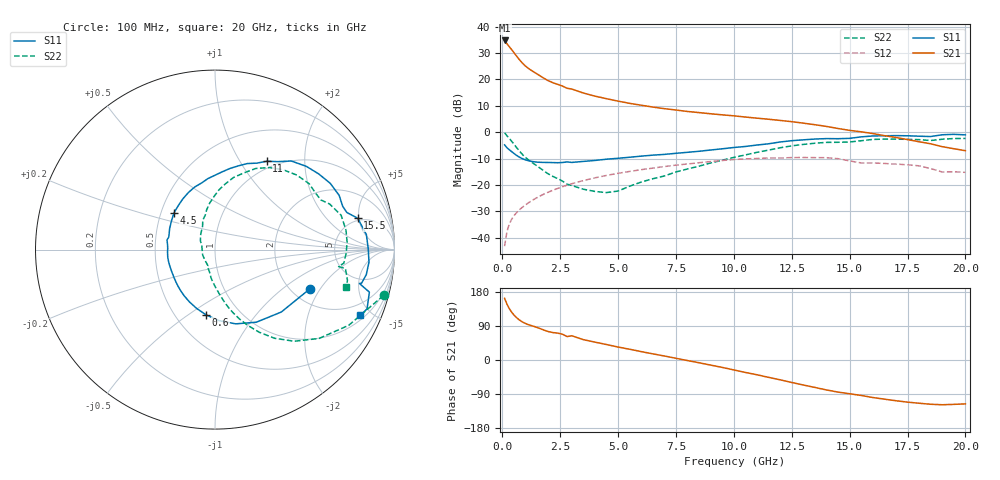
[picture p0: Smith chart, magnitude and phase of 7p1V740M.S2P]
! Infineon Technologies  Discrete & RF Semiconductors
! bfp620
! VCE =  1.7 V,  IC =  40 mA
! Common Emitter S-Parameters:  Sep 2002
# GHz  S  MA  R  50
!  f  S11  S21  S12  S22
! GHz  MAG  ANG  MAG  ANG  MAG  ANG  MAG  ANG
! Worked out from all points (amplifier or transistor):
!   59 points, 100 MHz to 20 GHz, reference 50 ohm
!   highest |S21| = 34.8 dB at 100 MHz (marker M1)
!   |S21| within 3 dB of that: start of sweep to 361.1 MHz
!   unconditionally stable (mu >= 1): 2.754 GHz to 2.94 GHz; 3.04 GHz to 9.824 GHz; 17.19 GHz to end of sweep
!   at 1 GHz: K = 0.82, MSG = 26.3 dB, |S12| = -27.6 dB
!   at 5.5 GHz: K = 1.04, MAG = 11.7 dB, |S12| = -14.9 dB
!   at 20 GHz: K = 1.29, MAG = 0.9 dB, |S12| = -15.2 dB
!   S11 on the Smith chart (normalised r, x): 100 MHz: 2.51, -1.62; 600 MHz: 0.70, -0.59; 4.5 GHz: 0.58, +0.27; 11 GHz: 0.90, +1.31; 15.5 GHz: 4.65, +4.82; 20 GHz: 1.23, -4.31
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0.1  0.5736 -22.2  54.75 162.6  0.0069 82.4  0.9735 -15.2
0.2  0.5073 -43.3  47.49 147.6  0.013 73.4  0.8564 -29.5
0.3  0.4654 -60.4  41.88 135.9  0.018 69.3  0.7622 -40.5
0.4  0.4295 -74.4  36.89 126.6  0.0222 66.8  0.6757 -49.1
0.5  0.3964 -86.7  32.34 119.0  0.0259 65.0  0.5952 -56.1
0.6  0.3674 -97.6  28.3 112.7  0.0292 63.8  0.5228 -61.8
0.7  0.3435 -107.3  24.85 107.4  0.0325 63.0  0.4603 -66.6
0.9  0.31 -123.4  19.74 99.3  0.0387 62.0  0.3664 -74.0
1.1  0.2899 -135.2  16.53 93.9  0.0449 61.4  0.3055 -79.0
1.3  0.2776 -144.5  14.4 89.9  0.0511 60.8  0.2634 -82.8
2  0.2664 -171.3  9.382 74.8  0.0733 56.9  0.1606 -97.6
2.8  0.273 168.7  6.79 61.9  0.0989 50.8  0.1031 -115.0
3  0.2668 164.9  6.574 64.0  0.1052 49.1  0.0975 -114.0
3.5  0.2789 154.9  5.517 53.7  0.1209 44.6  0.0829 -130.8
4.5  0.3073 137.9  4.309 40.8  0.1513 35.4  0.0716 -178.7
7  0.3789 101.3  2.79 10.6  0.2227 11.2  0.1477 117.9
10.5  0.5356 64.1  1.935 -32.9  0.3112 -28.3  0.3704 81.1
11  0.5701 59.7  1.842 -39.0  0.3171 -33.8  0.4149 75.6
13.5  0.7407 29.9  1.385 -72.4  0.3292 -64.7  0.6168 42.3
15.5  0.8141 12.4  1.015 -93.6  0.2608 -86.9  0.6873 21.7
17  0.8607 -4.7  0.793 -107.5  0.2483 -96.5  0.7373 3.1
20  0.8892 -24.3  0.445 -115.8  0.1732 -106.4  0.76 -15.8
